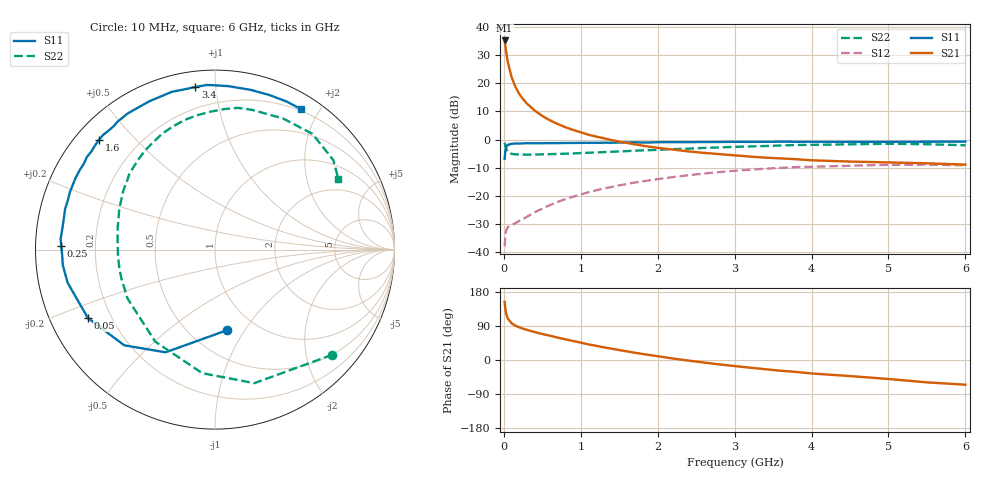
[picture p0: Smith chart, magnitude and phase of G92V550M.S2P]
! SIEMENS Small Signal Semiconductors
! BFG235
! Si NPN RF Bipolar Junction Transistor in SOT223
! VCE = 2.5 V  IC = 50 mA
! Common Emitter S-Parameters:  July  1994
# GHz  S  MA  R  50
!  f  S11  S21  S12  S22
! GHz  MAG  ANG  MAG  ANG  MAG  ANG  MAG  ANG
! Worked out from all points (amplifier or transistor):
!   40 points, 10 MHz to 6 GHz, reference 50 ohm
!   highest |S21| = 35.2 dB at 10 MHz (marker M1)
!   |S21| within 3 dB of that: start of sweep to 24.91 MHz
!   unconditionally stable (mu >= 1): 490.1 MHz to 1.482 GHz
!   at 200 MHz: K = 0.68, MSG = 22.5 dB, |S12| = -28.8 dB
!   at 1.5 GHz: K = 1.00, MSG = 7.8 dB, |S12| = -16.3 dB
!   at 6 GHz: K = 0.93, MSG = 0.1 dB, |S12| = -9.2 dB
!   S11 on the Smith chart (normalised r, x): 10 MHz: 0.74, -0.84; 50 MHz: 0.12, -0.25; 250 MHz: 0.08, +0.01; 1.6 GHz: 0.07, +0.40; 3.4 GHz: 0.08, +0.88; 6 GHz: 0.18, +1.78
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0.01  0.4547 -81.8  57.51 153.4  0.0128 64.9  0.8777 -41.9
0.02  0.6351 -115.7  45.64 134.7  0.0205 49.0  0.7758 -73.6
0.03  0.735 -133.5  36.16 122.7  0.0242 39.4  0.692 -95.9
0.05  0.8042 -151.7  24.26 109.8  0.0278 30.7  0.6113 -123.0
0.1  0.8415 -167.3  12.89 96.9  0.0304 29.0  0.5584 -150.9
0.15  0.8524 -174.2  8.654 90.6  0.0328 32.7  0.5458 -162.4
0.2  0.852 -177.9  6.476 86.3  0.0361 36.4  0.5434 -168.9
0.25  0.8567 178.7  5.22 82.6  0.0391 40.1  0.541 -173.3
0.3  0.8622 176.2  4.359 79.6  0.0426 43.0  0.5413 -176.9
0.4  0.8583 171.6  3.284 73.8  0.051 47.2  0.5421 178.0
0.5  0.8605 167.8  2.623 68.6  0.0594 50.0  0.5459 173.9
0.6  0.8654 164.8  2.195 64.1  0.0687 51.3  0.5507 170.2
0.7  0.865 161.1  1.893 59.0  0.0781 52.0  0.5564 166.9
0.9  0.8706 155.5  1.484 50.2  0.0966 50.6  0.5675 161.0
1.1  0.8743 149.2  1.221 41.2  0.116 48.7  0.5835 155.2
1.6  0.8899 136.6  0.871 22.8  0.1627 40.2  0.6232 141.5
2.2  0.9011 122.8  0.664 3.8  0.2159 27.8  0.676 125.2
3.2  0.909 101.2  0.499 -20.3  0.2918 4.5  0.7544 97.8
3.4  0.9124 96.9  0.477 -24.3  0.3035 -0.3  0.7688 91.9
4.5  0.912 77.4  0.407 -42.4  0.3425 -25.6  0.8232 62.6
5.5  0.9164 64.3  0.379 -59.0  0.3591 -47.5  0.8267 37.1
6  0.9181 58.4  0.359 -65.2  0.3485 -55.7  0.7916 29.8
